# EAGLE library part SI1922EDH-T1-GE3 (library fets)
MOSFET 2N-CH 20V 1.3A SOT-363
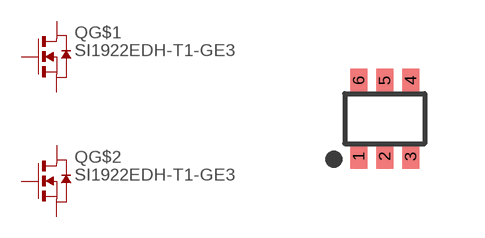
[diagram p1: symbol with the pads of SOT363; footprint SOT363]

Designator prefix Q; gates G$1=N_MOSFET G$2=N_MOSFET

## SI1922EDH-T1-GE3 (DIGIKEY: SI1922EDH-T1-GE3CT-ND; MANUFACTURER: Vishay Siliconix; MPN: SI1922EDH-T1-GE3)  [SOT363]
1  G$1:S  pas
2  G$1:G  pas
3  G$2:D  pas
4  G$2:S  pas
5  G$2:G  pas
6  G$1:D  pas

## Footprint SOT363 (pad centres in mm)
smd 0.42 x 0.6: 1 -0.65,-0.95; 2 0,-0.95; 3 0.65,-0.95; 4 0.65,0.95; 5 0,0.95; 6 -0.65,0.95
